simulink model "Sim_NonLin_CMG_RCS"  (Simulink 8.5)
settings: Solver=ode5  StartTime=0.0  StopTime=20000  FixedStep=Ts*2  RelTol=1e-3
InitFcn:
  | start
StopFcn:
  | Pl
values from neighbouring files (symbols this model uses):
  com_dir = com_dir/sqrt(com_dir'*com_dir)    [start.m]    (also in start1.m; start2.m; start3.m)
  d2r = pi/180    (= 0.0174532925199)    [start.m]    (also in Dead_Band_DF.m; start1.m; start2.m; start3.m)
  ini = [wbo; atto; Hco]    [start.m]    (also in start1.m; start2.m; start3.m)
  J = [0.119416e9, -0.476e7,   -0.1216e7;     -0.476e7,     0.40408e8, -0.30121e6;     -0.1216e7,   -0.30121e6,  0.110166e9]    [start.m]    (also in start1.m; start2.m; start3.m)
  KshC = 2*Wdot_Lim_CMG/WlimC    [start.m]    (also in start1.m; start2.m; start3.m)
  KshR = 2*Wdot_Lim_RCS/WlimR    [start.m]    (also in start1.m; start2.m; start3.m)
  nt = 12    [start.m]    (also in start1.m; start2.m; start3.m)
  omg = 20*wo    (= 0.022)    [start.m]    (also in start1.m; start2.m; start3.m)
  r2d = 180/pi    (= 57.2957795131)    [start.m]    (also in start1.m; start2.m; start3.m)
  thecmd = 3    [start.m]    (also in start1.m = 0.1; start2.m = 20; start3.m = 20)
  Wdot_Lim_CMG = 0.0001*d2r    (= 1.74532925199e-06)    [start.m]    (also in start1.m; start2.m; start3.m)
  Wdot_Lim_RCS = 0.02*d2r    (= 0.000349065850399)    [start.m]    (also in start1.m; start2.m; start3.m)
  Wlim_CMG = 0.01*d2r    (= 0.000174532925199)    [start.m]    (also in start1.m; start2.m; start3.m)
  Wlim_RCS = 0.6*d2r    (= 0.010471975512)    [start.m]    (also in start1.m; start2.m; start3.m)
  wo = 0.0011    [start.m]    (also in start1.m; start2.m; start3.m)
  zeb = 0.95    [start.m]    (also in start1.m; start2.m; start3.m)
undefined symbols (not defined in the file or in its folder): Phase_Plane, Rigbod_Dynam_LVLH, Torq_Lim, Wlim

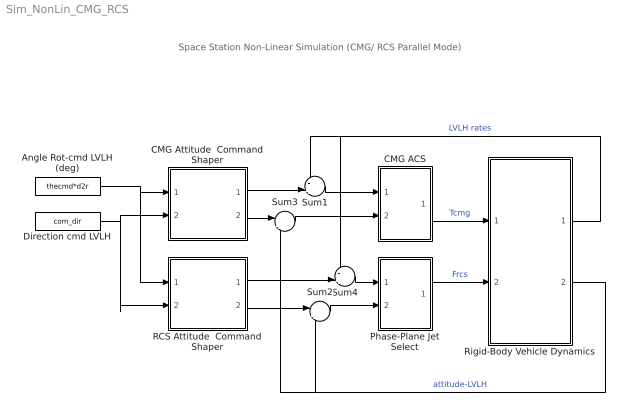
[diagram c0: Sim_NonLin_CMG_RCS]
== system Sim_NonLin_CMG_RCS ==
  note: Space Station Non-Linear Simulation (CMG/ RCS Parallel Mode)
  Angle Rot-cmd LVLH (deg) : Constant  Value=thecmd*d2r
  CMG ACS : Subsystem
  CMG Attitude  Command Shaper : Subsystem
  Direction cmd LVLH : Constant  Value=com_dir
  Phase-Plane Jet Select : Subsystem
  RCS Attitude  Command Shaper : Subsystem
  Rigid-Body Vehicle Dynamics : Subsystem
  Sum1 : Sum  Inputs=-+|
  Sum2 : Sum  Inputs=|+-
  Sum3 : Sum  Inputs=|+-
  Sum4 : Sum  Inputs=-+|
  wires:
  Rigid-Body Vehicle Dynamics/2(atti-lv) -> Sum2/2, Sum3/2  "attitude-LVLH"
  Sum2/1 -> Phase-Plane Jet Select/2(atter)
  Rigid-Body Vehicle Dynamics/1(w-lv) -> Sum1/1, Sum4/1  "LVLH rates"
  Direction cmd LVLH/1 -> CMG Attitude  Command Shaper/2(dir), RCS Attitude  Command Shaper/2(dir)
  Angle Rot-cmd LVLH (deg)/1 -> CMG Attitude  Command Shaper/1(cmd), RCS Attitude  Command Shaper/1(cmd)
  Sum1/1 -> CMG ACS/1(wl)
  CMG Attitude  Command Shaper/1(w-cmd) -> Sum1/2
  CMG Attitude  Command Shaper/2(att-cmd) -> Sum3/1
  Sum3/1 -> CMG ACS/2(ater)
  RCS Attitude  Command Shaper/2(att-cmd) -> Sum2/1
  Phase-Plane Jet Select/1(f(i)) -> Rigid-Body Vehicle Dynamics/2(f(i))  "Frcs"
  Sum4/1 -> Phase-Plane Jet Select/1(rater)
  RCS Attitude  Command Shaper/1(w-cmd) -> Sum4/2
  CMG ACS/1(Tq) -> Rigid-Body Vehicle Dynamics/1(Tc)  "Tcmg"

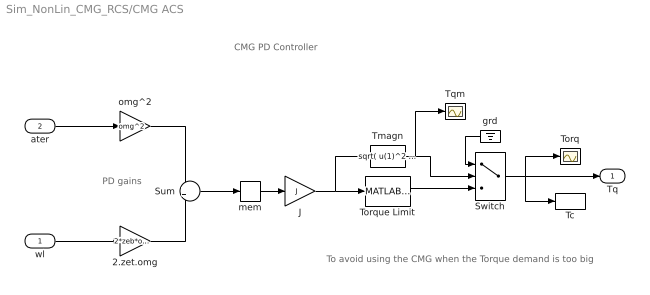
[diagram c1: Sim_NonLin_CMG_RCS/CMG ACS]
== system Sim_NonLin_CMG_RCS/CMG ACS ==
  note: CMG PD Controller
  note: PD gains
  note: To avoid using the CMG when the Torque demand is too big
  wl : Inport
  ater : Inport  Port=2  PortDimensions=3
  2.zet.omg : Gain  Gain=2*zeb*omg
  J : Gain  Gain=J  Multiplication=Matrix(K*u)
  Sum : Sum
  Switch : Switch  Threshold=800
  Tc : ToWorkspace  VariableName=Tcmg  SampleTime=-1
  Tmagn : Fcn  Expr=sqrt( u(1)^2 + u(2)^2 + u(3)^2 )
  Torq : Scope
  Torque Limit : MATLABFcn  MATLABFcn=Torq_Lim( u(1:3) )  OutputDimensions=3
  Tqm : Scope
  grd : Ground
  mem : Memory
  omg^2 : Gain  Gain=omg^2
  Tq : Outport
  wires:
  wl/1 -> 2.zet.omg/1
  Sum/1 -> mem/1
  2.zet.omg/1 -> Sum/2
  ater/1 -> omg^2/1
  omg^2/1 -> Sum/1
  J/1 -> Torque Limit/1, Tmagn/1
  mem/1 -> J/1
  Torque Limit/1 -> Switch/3
  Switch/1 -> Tq/1, Torq/1, Tc/1
  Tmagn/1 -> Switch/2, Tqm/1
  grd/1 -> Switch/1

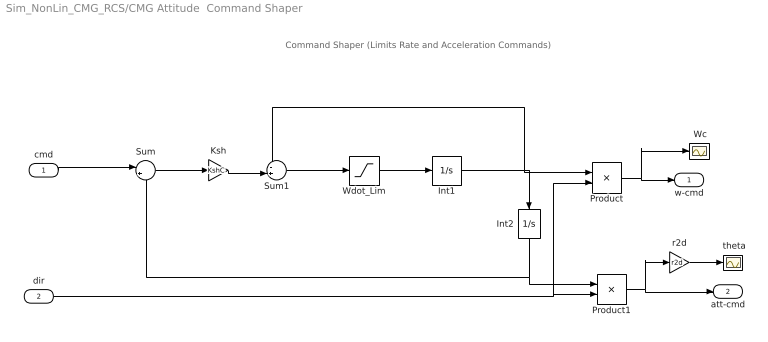
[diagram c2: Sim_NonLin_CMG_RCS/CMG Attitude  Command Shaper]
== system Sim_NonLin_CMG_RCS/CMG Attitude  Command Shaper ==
  note: Command Shaper (Limits Rate and Acceleration Commands)
  cmd : Inport  PortDimensions=1
  dir : Inport  Port=2  PortDimensions=3
  " Wc" : Scope
  " theta" : Scope
  Int1 : Integrator  LimitOutput=on  UpperSaturationLimit=Wlim_CMG  LowerSaturationLimit=-Wlim_CMG
  Int2 : Integrator  UpperSaturationLimit=Wlim  LowerSaturationLimit=-Wlim
  Ksh : Gain  Gain=KshC
  Product : Product
  Product1 : Product
  Sum : Sum  Inputs=|+-
  Sum1 : Sum  Inputs=-+|
  Wdot_Lim : Saturate  UpperLimit=Wdot_Lim_CMG  LowerLimit=-Wdot_Lim_CMG
  r2d : Gain  Gain=r2d
  w-cmd : Outport  PortDimensions=3
  att-cmd : Outport  Port=2  PortDimensions=3
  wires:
  Wdot_Lim/1 -> Int1/1
  Sum1/1 -> Wdot_Lim/1
  Int1/1 -> Product/1, Sum1/1, Int2/1
  Sum/1 -> Ksh/1
  Ksh/1 -> Sum1/2
  Int2/1 -> Sum/2, Product1/1
  cmd/1 -> Sum/1
  dir/1 -> Product/2, Product1/2
  r2d/1 -> " theta"/1
  Product/1 -> w-cmd/1, " Wc"/1
  Product1/1 -> att-cmd/1, r2d/1

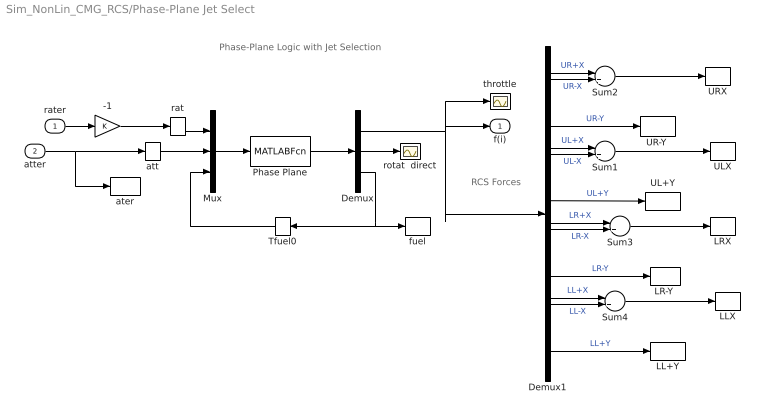
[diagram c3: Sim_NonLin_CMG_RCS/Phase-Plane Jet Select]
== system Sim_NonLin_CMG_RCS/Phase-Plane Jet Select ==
  note: Phase-Plane Logic with Jet Selection
  note: RCS Forces
  rater : Inport
  atter : Inport  Port=2
  -1 : Gain
  Demux : Demux  Outputs=[nt, 3,1]
  Demux1 : Demux  Outputs=nt
  LL+Y : ToWorkspace  VariableName=LLPY  SampleTime=-1
  LLX : ToWorkspace  VariableName=LLX  SampleTime=-1
  "LR-Y " : ToWorkspace  VariableName=LRNY  SampleTime=-1
  LRX : ToWorkspace  VariableName=LRX  SampleTime=-1
  Mux : Mux  Inputs="[3  3  1]"
  Phase Plane : MATLABFcn  MATLABFcn=Phase_Plane( u(1:3), u(4:6), u(7) )  OutputDimensions=nt + 4
  Sum{1..4} (4 alike) : Sum  Inputs=|++
  Tfuel0 : Memory
  UL+Y : ToWorkspace  VariableName=ULPY  SampleTime=-1
  ULX : ToWorkspace  VariableName=ULX  SampleTime=-1
  "UR-Y " : ToWorkspace  VariableName=URNY  SampleTime=-1
  URX : ToWorkspace  VariableName=URX  SampleTime=-1
  ater : ToWorkspace  VariableName=atter  SampleTime=-1
  att : Memory
  fuel : ToWorkspace  VariableName=Fuel  SampleTime=-1
  rat : Memory
  rotat  direct : Scope
  throttle : Scope
  f(i) : Outport
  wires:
  Demux/3 -> Tfuel0/1, fuel/1
  att/1 -> Mux/2
  atter/1 -> att/1, ater/1
  rater/1 -> -1/1
  Demux/2 -> rotat  direct/1
  Demux/1 -> f(i)/1, Demux1/1, throttle/1
  Tfuel0/1 -> Mux/3
  Phase Plane/1 -> Demux/1
  Mux/1 -> Phase Plane/1
  rat/1 -> Mux/1
  Demux1/1 -> Sum2/1  "UR+X"
  Demux1/2 -> Sum2/2  "UR-X"
  Sum2/1 -> URX/1
  Demux1/4 -> Sum1/1  "UL+X"
  Demux1/5 -> Sum1/2  "UL-X"
  Demux1/7 -> Sum3/1  "LR+X"
  Demux1/8 -> Sum3/2  "LR-X"
  Demux1/10 -> Sum4/1  "LL+X"
  Demux1/11 -> Sum4/2  "LL-X"
  Sum1/1 -> ULX/1
  Sum3/1 -> LRX/1
  Sum4/1 -> LLX/1
  Demux1/3 -> "UR-Y "/1  "UR-Y"
  Demux1/6 -> UL+Y/1  "UL+Y"
  Demux1/12 -> LL+Y/1  "LL+Y"
  Demux1/9 -> "LR-Y "/1  "LR-Y"
  -1/1 -> rat/1

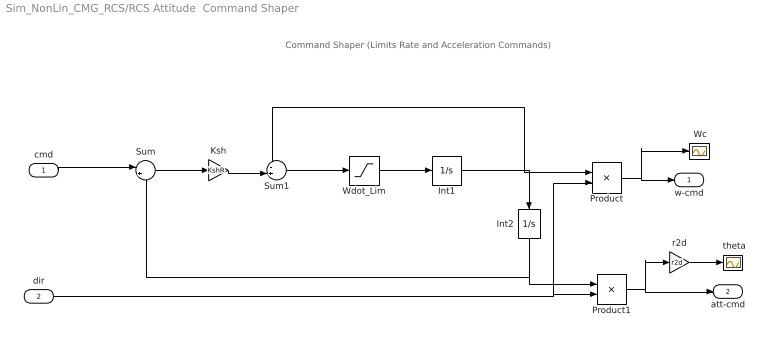
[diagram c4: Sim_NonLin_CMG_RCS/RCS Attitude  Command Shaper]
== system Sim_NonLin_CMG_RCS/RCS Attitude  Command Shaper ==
  note: Command Shaper (Limits Rate and Acceleration Commands)
  cmd : Inport  PortDimensions=1
  dir : Inport  Port=2  PortDimensions=3
  " Wc" : Scope
  " theta" : Scope
  Int1 : Integrator  LimitOutput=on  UpperSaturationLimit=Wlim_RCS  LowerSaturationLimit=-Wlim_RCS
  Int2 : Integrator  UpperSaturationLimit=Wlim  LowerSaturationLimit=-Wlim
  Ksh : Gain  Gain=KshR
  Product : Product
  Product1 : Product
  Sum : Sum  Inputs=|+-
  Sum1 : Sum  Inputs=-+|
  Wdot_Lim : Saturate  UpperLimit=Wdot_Lim_RCS  LowerLimit=-Wdot_Lim_RCS
  r2d : Gain  Gain=r2d
  w-cmd : Outport  PortDimensions=3
  att-cmd : Outport  Port=2  PortDimensions=3
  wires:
  Wdot_Lim/1 -> Int1/1
  Sum1/1 -> Wdot_Lim/1
  Int1/1 -> Product/1, Sum1/1, Int2/1
  Sum/1 -> Ksh/1
  Ksh/1 -> Sum1/2
  Int2/1 -> Sum/2, Product1/1
  cmd/1 -> Sum/1
  dir/1 -> Product/2, Product1/2
  r2d/1 -> " theta"/1
  Product/1 -> w-cmd/1, " Wc"/1
  Product1/1 -> att-cmd/1, r2d/1

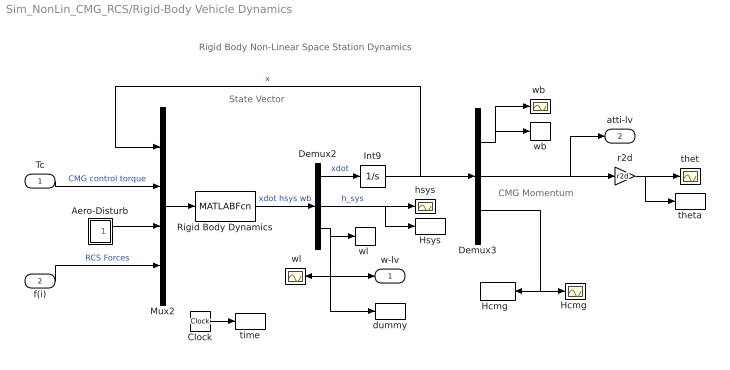
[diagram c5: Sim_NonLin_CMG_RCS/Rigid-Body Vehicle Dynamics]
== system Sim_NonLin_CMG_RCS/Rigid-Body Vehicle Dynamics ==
  note: Rigid Body Non-Linear Space Station Dynamics
  note: State Vector
  note: CMG Momentum
  Tc : Inport  PortDimensions=3
  f(i) : Inport  Port=2  PortDimensions=nt
  " wl" : Scope
  Aero-Disturb : Subsystem
  Clock : Clock
  Demux2 : Demux  Outputs=[9,3,3]
  Demux3 : Demux  Outputs=[3,3,3]
  "Hcmg " : Scope
  "Hcmg  " : ToWorkspace  VariableName=Hcmg  SampleTime=-1
  Hsys : ToWorkspace  VariableName=Hsys  SampleTime=-1
  Int9 : Integrator  InitialCondition=ini
  Mux2 : Mux  Inputs=[9, 3, 3, nt]
  Rigid Body Dynamics : MATLABFcn  MATLABFcn=Rigbod_Dynam_LVLH( u(1:9), u(10:12), u(13:15), u(16:15+nt) )  OutputDimensions=15
  dummy : ToWorkspace  VariableName=accel  SampleTime=-1
  hsys : Scope
  r2d : Gain  Gain=r2d
  thet : Scope
  theta : ToWorkspace  VariableName=theta  SampleTime=-1
  time : ToWorkspace  VariableName=time  SampleTime=-1
  wb : ToWorkspace  VariableName=wb  SampleTime=-1
  "wb " : Scope
  "wl " : ToWorkspace  VariableName=wl  SampleTime=-1
  w-lv : Outport
  atti-lv : Outport  Port=2
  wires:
  Rigid Body Dynamics/1 -> Demux2/1  "xdot hsys wb"
  Demux2/1 -> Int9/1  "xdot"
  Int9/1 -> Demux3/1, Mux2/1  "x"
  Tc/1 -> Mux2/2  "CMG control torque"
  Demux2/3 -> "wl "/1, w-lv/1, " wl"/1, dummy/1
  Demux2/2 -> hsys/1, Hsys/1  "h_sys"
  Demux3/2 -> r2d/1, atti-lv/1
  Demux3/3 -> "Hcmg  "/1, "Hcmg "/1
  f(i)/1 -> Mux2/4  "RCS Forces"
  r2d/1 -> thet/1, theta/1
  Clock/1 -> time/1
  Mux2/1 -> Rigid Body Dynamics/1
  Demux3/1 -> "wb "/1, wb/1
  Aero-Disturb/1(Td) -> Mux2/3

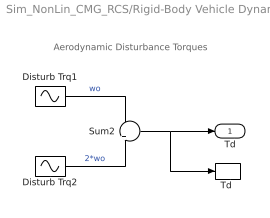
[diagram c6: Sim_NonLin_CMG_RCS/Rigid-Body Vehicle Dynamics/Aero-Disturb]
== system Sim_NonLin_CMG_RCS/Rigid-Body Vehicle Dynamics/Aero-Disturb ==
  note: Aerodynamic Disturbance Torques
  Disturb Trq1 : Sin  Amplitude=[1, 3, 1]  Bias="[1  8  1]"  Frequency=[wo, wo, wo]  SampleTime=0
  Disturb Trq2 : Sin  Amplitude=[1, 1, 1]*0.5  Frequency=[wo, wo, wo]*2  SampleTime=0
  Sum2 : Sum  Inputs=+|+
  "Td " : ToWorkspace  VariableName=Td  SampleTime=-1
  Td : Outport
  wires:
  Disturb Trq1/1 -> Sum2/1  "wo"
  Sum2/1 -> Td/1, "Td "/1
  Disturb Trq2/1 -> Sum2/2  "2*wo"
